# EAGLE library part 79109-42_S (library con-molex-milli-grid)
RECEPTACAL
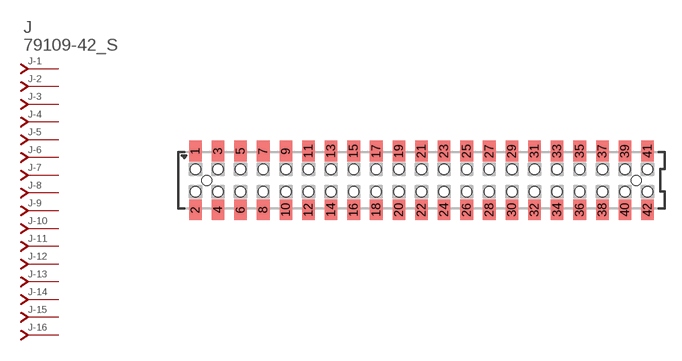
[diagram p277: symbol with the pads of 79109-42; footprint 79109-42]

Designator prefix J; gates -1=J-NV -2=J-N -3=J-N -4=J-N -5=J-N -6=J-N -7=J-N -8=J-N -9=J-N -10=J-N -11=J-N -12=J-N -13=J-N -14=J-N -15=J-N -16=J-N -17=J-N -18=J-N -19=J-N -20=J-N -21=J-N -22=J-N -23=J-N -24=J-N -25=J-N -26=J-N -27=J-N -28=J-N -29=J-N -30=J-N -31=J-N -32=J-N -33=J-N -34=J-N -35=J-N -36=J-N -37=J-N -38=J-N -39=J-N -40=J-N -41=J-N -42=J-N

## 79109-42_S  [79109-42]
1  -1:J  pas
2  -2:J  pas
3  -3:J  pas
4  -4:J  pas
5  -5:J  pas
6  -6:J  pas
7  -7:J  pas
8  -8:J  pas
9  -9:J  pas
10  -10:J  pas
11  -11:J  pas
12  -12:J  pas
13  -13:J  pas
14  -14:J  pas
15  -15:J  pas
16  -16:J  pas
17  -17:J  pas
18  -18:J  pas
19  -19:J  pas
20  -20:J  pas
21  -21:J  pas
22  -22:J  pas
23  -23:J  pas
24  -24:J  pas
25  -25:J  pas
26  -26:J  pas
27  -27:J  pas
28  -28:J  pas
29  -29:J  pas
30  -30:J  pas
31  -31:J  pas
32  -32:J  pas
33  -33:J  pas
34  -34:J  pas
35  -35:J  pas
36  -36:J  pas
37  -37:J  pas
38  -38:J  pas
39  -39:J  pas
40  -40:J  pas
41  -41:J  pas
42  -42:J  pas

## Footprint 79109-42 (pad centres in mm)
RECEPTACAL SMD Dual Row, Vertical, Pass-Thru
smd 1.12 x 1.83: 1 -20,2.6; 2 -20,-2.6; 3 -18,2.6; 4 -18,-2.6; 5 -16,2.6; 6 -16,-2.6; 7 -14,2.6; 8 -14,-2.6; 9 -12,2.6; 10 -12,-2.6; 11 -10,2.6; 12 -10,-2.6; 13 -8,2.6; 14 -8,-2.6; 15 -6,2.6; 16 -6,-2.6; 17 -4,2.6; 18 -4,-2.6; 19 -2,2.6; 20 -2,-2.6; 21 0,2.6; 22 0,-2.6; 23 2,2.6; 24 2,-2.6; 25 4,2.6; 26 4,-2.6; 27 6,2.6; 28 6,-2.6; 29 8,2.6; 30 8,-2.6; 31 10,2.6; 32 10,-2.6; 33 12,2.6; 34 12,-2.6; 35 14,2.6; 36 14,-2.6; 37 16,2.6; 38 16,-2.6; 39 18,2.6; 40 18,-2.6; 41 20,2.6; 42 20,-2.6
hole 0.914 at -19,0
hole 0.914 at -20,1
hole 0.914 at -20,-1
hole 0.914 at -18,-1
hole 0.914 at -18,1
hole 0.914 at -16,-1
hole 0.914 at -16,1
hole 0.914 at 19,0
hole 0.914 at -14,1
hole 0.914 at -14,-1
hole 0.914 at -12,1
hole 0.914 at -12,-1
hole 0.914 at -10,1
hole 0.914 at -10,-1
hole 0.914 at -8,1
hole 0.914 at -8,-1
hole 0.914 at -6,-1
hole 0.914 at -6,1
hole 0.914 at -4,1
hole 0.914 at -4,-1
hole 0.914 at -2,1
hole 0.914 at -2,-1
hole 0.914 at 0,1
hole 0.914 at 0,-1
hole 0.914 at 2,-1
hole 0.914 at 2,1
hole 0.914 at 4,1
hole 0.914 at 6,1
hole 0.914 at 8,1
hole 0.914 at 4,-1
hole 0.914 at 6,-1
hole 0.914 at 8,-1
hole 0.914 at 10,-1
hole 0.914 at 12,-1
hole 0.914 at 14,-1
hole 0.914 at 16,-1
hole 0.914 at 18,-1
hole 0.914 at 10,1
hole 0.914 at 12,1
hole 0.914 at 14,1
hole 0.914 at 16,1
hole 0.914 at 18,1
hole 0.914 at 20,-1
hole 0.914 at 20,1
